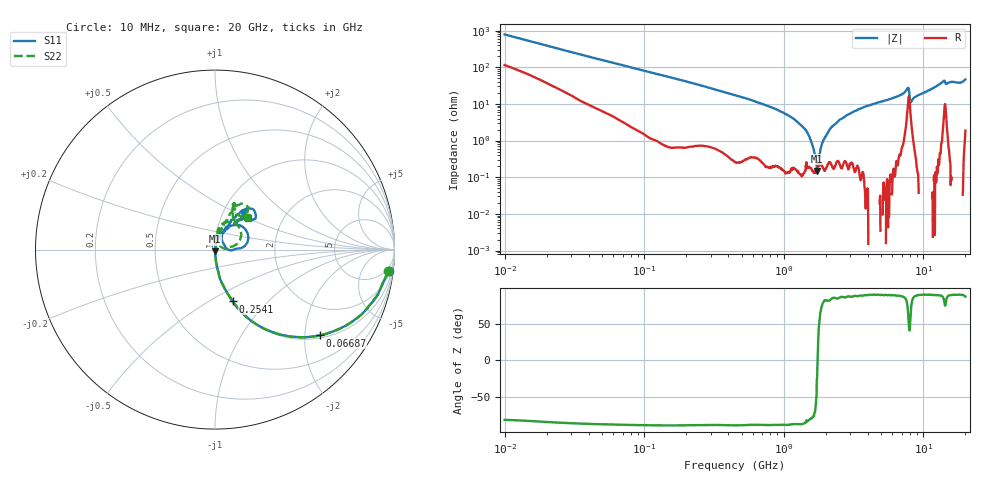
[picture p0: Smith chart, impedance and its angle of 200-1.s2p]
!Keysight Technologies,P5008B,MY61100088,A.16.20.02
!Date: Monday, May 27, 2024 17:24:07
!Correction: S11(C* 2-Port  )
!S21(C* 2-Port  )
!S12(C* 2-Port  )
!S22(C* 2-Port  )
!S2P File: Measurements: S11, S21, S12, S22:Log Frequency Sweep
# Hz S  dB  R 50
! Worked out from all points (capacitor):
!   1601 points, 10 MHz to 20 GHz, reference 50 ohm
!   read as one part in series: C = 20.5 pF near 10.39 MHz
!   lowest |Z| = 147 mohm at 1.732 GHz (marker M1)
!   series resonance near 1.746 GHz, so ESL is about 400 pH
!   S11 on the Smith chart (normalised r, x): 10 MHz: 3, -16; 66.87 MHz: 1.07, -2.38; 254.1 MHz: 1.01, -0.65; 20 GHz: 1.34, +0.50
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1e7  -0.21 -7.1  -18.12 74.5  -18.13 74.6  -0.23 -7.0
3.555162e7  -0.98 -23.8  -7.83 63.1  -7.84 63.1  -0.99 -23.9
6.687403e7  -2.45 -39.3  -3.95 48.9  -3.96 48.9  -2.45 -39.4
1.263918e8  -5.40 -56.8  -1.57 32.5  -1.58 32.5  -5.39 -56.8
2.540978e8  -10.30 -71.1  -0.48 17.6  -0.49 17.6  -10.31 -71.1
4.472136e8  -15.25 -79.7  -0.16 9.7  -0.16 9.7  -15.24 -79.7
1.118669e9  -26.02 -86.6  -0.02 2.3  -0.03 2.2  -25.99 -85.1
1.425352e9  -31.51 -87.7  -0.00 0.7  -0.02 0.7  -31.29 -81.5
1.589917e9  -36.58 -87.3  -0.00 0.1  -0.01 0.1  -35.63 -75.4
1.731853e9  -39.86 -83.2  0.00 -0.5  -0.01 -0.5  -41.16 -69.4
1.859765e9  -54.32 -38.2  0.00 -0.9  -0.01 -0.9  -43.64 -25.6
1.92265e9  -55.42 65.6  0.00 -1.1  -0.01 -1.1  -45.33 -2.3
2.154843e9  -38.63 75.8  0.00 -1.8  -0.01 -1.8  -38.49 51.6
2.496738e9  -32.41 80.5  0.00 -2.8  -0.01 -2.8  -32.60 70.0
3.685962e9  -25.28 87.3  -0.00 -5.9  -0.01 -5.9  -24.35 74.8
5.652411e9  -21.21 78.0  -0.02 -10.3  -0.03 -10.3  -21.25 79.9
7.624508e9  -14.82 49.4  -0.47 -17.5  -0.48 -17.5  -15.37 64.1
8.384452e9  -24.69 40.5  -0.08 -12.6  -0.09 -12.6  -26.26 78.5
1.367661e10  -11.04 53.0  -0.39 -28.1  -0.40 -28.1  -11.13 63.0
1.61506e10  -11.18 51.1  -0.27 -29.7  -0.28 -29.7  -11.23 67.5
1.836088e10  -14.72 53.1  -0.07 -34.2  -0.08 -34.3  -14.66 57.0
2e10  -11.92 44.0  -0.38 -39.8  -0.39 -39.9  -11.83 45.7
